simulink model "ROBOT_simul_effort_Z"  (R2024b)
settings: Solver=VariableStepAuto  StartTime=0.0  StopTime=5  RelTol=1e-3
undefined symbols (not defined in the file): a, ARRIERE_Defaut_sldprt, avant01_Defaut_sldprt, avant02_Defaut_sldprt, avant03_Defaut_sldprt, avant1_Defaut_sldprt, AXE, BASE_Defaut_sldprt, BIELLE, BIELLE_Defaut_sldprt, BRAS_Defaut_sldprt, bras_Defaut_sldprt, C_Realiste_sldprt, CABLE_Defaut_sldprt, cable_Defaut_sldprt, CACHE_Defaut_sldprt, CARTE, carte_Defaut_sldprt, CARTER, carter, CHC, CODEUR_Defaut_sldprt, cruciforme, cylindrique, deg, Drive, Fichiers, Fichiers_Matlab_sujetA, FIXATION, fixation_Defaut_sldprt, H, HEXAGONALE_Defaut_sldprt, joint_Defaut_sldprt, kg, m, M4, M4_Defaut_sldprt, manette1_Defaut_sldprt, manette2_Defaut_sldprt, MATLAB, Matlab, matlab_Defaut_sldprt, mm, modif, MOTEUR_Defaut_sldprt, N, NEZ_Defaut_sldprt, nom, palier, PARALLELOGRAMME_Defaut_sldprt, petite, plaque, rad, Ressort, Rondelle, ROTOR_Defaut_sldprt, s, SET, simple, socle_Defaut_sldprt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
libraries: sm_lib x463, fl_lib x45, nesl_utility x27, simulink x2
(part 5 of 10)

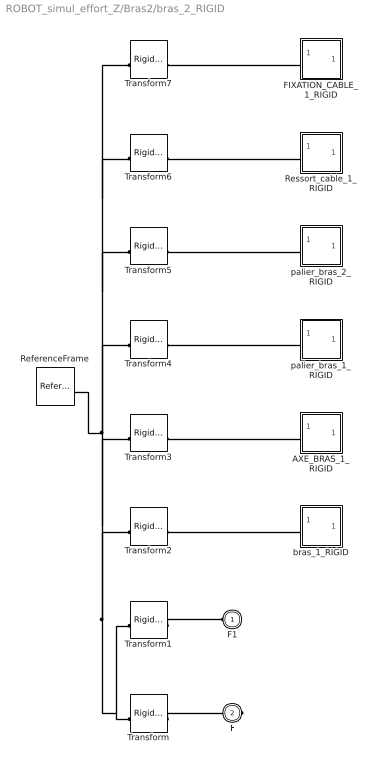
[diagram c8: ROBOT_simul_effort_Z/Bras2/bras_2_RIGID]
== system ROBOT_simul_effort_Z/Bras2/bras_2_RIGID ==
  AXE_BRAS_1_RIGID : Subsystem
  FIXATION_CABLE_1_RIGID : Subsystem
  ReferenceFrame : sm_lib/Frames and Transforms/Reference Frame
  Ressort_cable_1_RIGID : Subsystem
  Transform : sm_lib/Frames and Transforms/Rigid Transform  RotationMethod=ArbitraryAxis  FollAlignAxisA=+X  BaseAlignAxisA=+Y  FollAlignAxisB=+Y  BaseAlignAxisB=+Z  RotationStandardAxis=+Z  RotationAngle=2.0943951023931953  RotationAngleUnits=rad  RotationArbitraryAxis=[0.57735026918962584 0.57735026918962562 0.57735026918962584]  RotationSequenceAxes=FollowerAxes  RotationSequence=XYX  RotationSequenceAngles=[0 0 0]  RotationSequenceAnglesUnits=deg  RotationMatrix=[1 0 0; 0 1 0; 0 0 1]  Quaternion=[1 0 0 0]  TranslationMethod=Cartesian  TranslationCartesianOffset=[-176.59192436800635 99.825618202078147 -20.98098974470366]  TranslationCartesianOffsetUnits=mm  TranslationStandardAxis=+Z  TranslationStandardOffset=0  TranslationStandardOffsetUnits=mm  TranslationROffset=0  TranslationROffsetUnits=m  TranslationThetaOffset=0  TranslationThetaOffsetUnits=deg  TranslationZOffset=0  TranslationZOffsetUnits=m
  Transform1 : sm_lib/Frames and Transforms/Rigid Transform  RotationMethod=ArbitraryAxis  FollAlignAxisA=+X  BaseAlignAxisA=+Y  FollAlignAxisB=+Y  BaseAlignAxisB=+Z  RotationStandardAxis=+Z  RotationAngle=2.0943951023931948  RotationAngleUnits=rad  RotationArbitraryAxis=[0.57735026918962573 0.57735026918962562 0.57735026918962595]  RotationSequenceAxes=FollowerAxes  RotationSequence=XYX  RotationSequenceAngles=[0 0 0]  RotationSequenceAnglesUnits=deg  RotationMatrix=[1 0 0; 0 1 0; 0 0 1]  Quaternion=[1 0 0 0]  TranslationMethod=Cartesian  TranslationCartesianOffset=[-252.36832285678628 39.825618202076186 -20.980989744713362]  TranslationCartesianOffsetUnits=mm  TranslationStandardAxis=+Z  TranslationStandardOffset=0  TranslationStandardOffsetUnits=mm  TranslationROffset=0  TranslationROffsetUnits=m  TranslationThetaOffset=0  TranslationThetaOffsetUnits=deg  TranslationZOffset=0  TranslationZOffsetUnits=m
  Transform2 : sm_lib/Frames and Transforms/Rigid Transform  RotationMethod=ArbitraryAxis  FollAlignAxisA=+X  BaseAlignAxisA=+Y  FollAlignAxisB=+Y  BaseAlignAxisB=+Z  RotationStandardAxis=+Z  RotationAngle=1.5707963267948968  RotationAngleUnits=rad  RotationArbitraryAxis=[9.841111005584301e-17 -1 -9.841111005584301e-17]  RotationSequenceAxes=FollowerAxes  RotationSequence=XYX  RotationSequenceAngles=[0 0 0]  RotationSequenceAnglesUnits=deg  RotationMatrix=[1 0 0; 0 1 0; 0 0 1]  Quaternion=[1 0 0 0]  TranslationMethod=Cartesian  TranslationCartesianOffset=[-166.59192436800635 39.825618202078161 -20.98098974470367]  TranslationCartesianOffsetUnits=mm  TranslationStandardAxis=+Z  TranslationStandardOffset=0  TranslationStandardOffsetUnits=mm  TranslationROffset=0  TranslationROffsetUnits=m  TranslationThetaOffset=0  TranslationThetaOffsetUnits=deg  TranslationZOffset=0  TranslationZOffsetUnits=m
  Transform3 : sm_lib/Frames and Transforms/Rigid Transform  RotationMethod=ArbitraryAxis  FollAlignAxisA=+X  BaseAlignAxisA=+Y  FollAlignAxisB=+Y  BaseAlignAxisB=+Z  RotationStandardAxis=+Z  RotationAngle=1.5707963267948968  RotationAngleUnits=rad  RotationArbitraryAxis=[-9.841111005584301e-17 1 -9.841111005584301e-17]  RotationSequenceAxes=FollowerAxes  RotationSequence=XYX  RotationSequenceAngles=[0 0 0]  RotationSequenceAnglesUnits=deg  RotationMatrix=[1 0 0; 0 1 0; 0 0 1]  Quaternion=[1 0 0 0]  TranslationMethod=Cartesian  TranslationCartesianOffset=[-166.59192436800635 39.825618202078161 -20.98098974470367]  TranslationCartesianOffsetUnits=mm  TranslationStandardAxis=+Z  TranslationStandardOffset=0  TranslationStandardOffsetUnits=mm  TranslationROffset=0  TranslationROffsetUnits=m  TranslationThetaOffset=0  TranslationThetaOffsetUnits=deg  TranslationZOffset=0  TranslationZOffsetUnits=m
  Transform4 : sm_lib/Frames and Transforms/Rigid Transform  RotationMethod=None  FollAlignAxisA=+X  BaseAlignAxisA=+Y  FollAlignAxisB=+Y  BaseAlignAxisB=+Z  RotationStandardAxis=+Z  RotationAngle=0  RotationAngleUnits=deg  RotationArbitraryAxis=[0 0 1]  RotationSequenceAxes=FollowerAxes  RotationSequence=XYX  RotationSequenceAngles=[0 0 0]  RotationSequenceAnglesUnits=deg  RotationMatrix=[1 0 0; 0 1 0; 0 0 1]  Quaternion=[1 0 0 0]  TranslationMethod=None  TranslationCartesianOffset=[0 0 0]  TranslationCartesianOffsetUnits=m  TranslationStandardAxis=+Z  TranslationStandardOffset=0  TranslationStandardOffsetUnits=m  TranslationROffset=0  TranslationROffsetUnits=m  TranslationThetaOffset=0  TranslationThetaOffsetUnits=deg  TranslationZOffset=0  TranslationZOffsetUnits=m
  Transform5 : sm_lib/Frames and Transforms/Rigid Transform  RotationMethod=ArbitraryAxis  FollAlignAxisA=+X  BaseAlignAxisA=+Y  FollAlignAxisB=+Y  BaseAlignAxisB=+Z  RotationStandardAxis=+Z  RotationAngle=3.1415926535897931  RotationAngleUnits=rad  RotationArbitraryAxis=[5.9196876012963212e-17 0.83121877946981937 -0.55594544755461739]  RotationSequenceAxes=FollowerAxes  RotationSequence=XYX  RotationSequenceAngles=[0 0 0]  RotationSequenceAnglesUnits=deg  RotationMatrix=[1 0 0; 0 1 0; 0 0 1]  Quaternion=[1 0 0 0]  TranslationMethod=Cartesian  TranslationCartesianOffset=[-333.18384873601269 5.2270863233389981 7.8152493791980318]  TranslationCartesianOffsetUnits=mm  TranslationStandardAxis=+Z  TranslationStandardOffset=0  TranslationStandardOffsetUnits=mm  TranslationROffset=0  TranslationROffsetUnits=m  TranslationThetaOffset=0  TranslationThetaOffsetUnits=deg  TranslationZOffset=0  TranslationZOffsetUnits=m
  Transform6 : sm_lib/Frames and Transforms/Rigid Transform  RotationMethod=ArbitraryAxis  FollAlignAxisA=+X  BaseAlignAxisA=+Y  FollAlignAxisB=+Y  BaseAlignAxisB=+Z  RotationStandardAxis=+Z  RotationAngle=1.5707963267948968  RotationAngleUnits=rad  RotationArbitraryAxis=[1 -9.841111005584301e-17 9.8411110055842801e-17]  RotationSequenceAxes=FollowerAxes  RotationSequence=XYX  RotationSequenceAngles=[0 0 0]  RotationSequenceAnglesUnits=deg  RotationMatrix=[1 0 0; 0 1 0; 0 0 1]  Quaternion=[1 0 0 0]  TranslationMethod=Cartesian  TranslationCartesianOffset=[-166.59192436800635 17.1829411352671 -24.980989744703674]  TranslationCartesianOffsetUnits=mm  TranslationStandardAxis=+Z  TranslationStandardOffset=0  TranslationStandardOffsetUnits=mm  TranslationROffset=0  TranslationROffsetUnits=m  TranslationThetaOffset=0  TranslationThetaOffsetUnits=deg  TranslationZOffset=0  TranslationZOffsetUnits=m
  Transform7 : sm_lib/Frames and Transforms/Rigid Transform  RotationMethod=ArbitraryAxis  FollAlignAxisA=+X  BaseAlignAxisA=+Y  FollAlignAxisB=+Y  BaseAlignAxisB=+Z  RotationStandardAxis=+Z  RotationAngle=1.0159852938148253  RotationAngleUnits=rad  RotationArbitraryAxis=[-1 0 -1.1577777653628589e-16]  RotationSequenceAxes=FollowerAxes  RotationSequence=XYX  RotationSequenceAngles=[0 0 0]  RotationSequenceAnglesUnits=deg  RotationMatrix=[1 0 0; 0 1 0; 0 0 1]  Quaternion=[1 0 0 0]  TranslationMethod=Cartesian  TranslationCartesianOffset=[-172.59192436800635 90.586314327933934 3.4188407632840172]  TranslationCartesianOffsetUnits=mm  TranslationStandardAxis=+Z  TranslationStandardOffset=0  TranslationStandardOffsetUnits=mm  TranslationROffset=0  TranslationROffsetUnits=m  TranslationThetaOffset=0  TranslationThetaOffsetUnits=deg  TranslationZOffset=0  TranslationZOffsetUnits=m
  bras_1_RIGID : Subsystem
  palier_bras_1_RIGID : Subsystem
  palier_bras_2_RIGID : Subsystem
  F1 : PMIOPort  Side=Left
  F : PMIOPort  Port=2  Side=Right
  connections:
  Transform/LConn1 -- ReferenceFrame/RConn1 -- Transform6/LConn1 -- Transform7/LConn1 -- Transform5/LConn1 -- Transform4/LConn1 -- Transform3/LConn1 -- Transform2/LConn1 -- Transform1/LConn1
  Transform/RConn1 -- F/RConn1
  Transform1/RConn1 -- F1/RConn1
  Transform2/RConn1 -- bras_1_RIGID/LConn1
  AXE_BRAS_1_RIGID/LConn1 -- Transform3/RConn1
  Transform4/RConn1 -- palier_bras_1_RIGID/LConn1
  Transform5/RConn1 -- palier_bras_2_RIGID/LConn1
  Ressort_cable_1_RIGID/LConn1 -- Transform6/RConn1
  FIXATION_CABLE_1_RIGID/LConn1 -- Transform7/RConn1

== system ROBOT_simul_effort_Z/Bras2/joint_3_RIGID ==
  AXE_BRAS_1_RIGID : Subsystem
  ReferenceFrame : sm_lib/Frames and Transforms/Reference Frame
  Transform : sm_lib/Frames and Transforms/Rigid Transform  RotationMethod=ArbitraryAxis  FollAlignAxisA=+X  BaseAlignAxisA=+Y  FollAlignAxisB=+Y  BaseAlignAxisB=+Z  RotationStandardAxis=+Z  RotationAngle=2.0943951023931953  RotationAngleUnits=rad  RotationArbitraryAxis=[0.57735026918962584 0.57735026918962584 0.57735026918962584]  RotationSequenceAxes=FollowerAxes  RotationSequence=XYX  RotationSequenceAngles=[0 0 0]  RotationSequenceAnglesUnits=deg  RotationMatrix=[1 0 0; 0 1 0; 0 0 1]  Quaternion=[1 0 0 0]  TranslationMethod=Cartesian  TranslationCartesianOffset=[-182.62772197331239 126.3991346976174 -143.1183707091507]  TranslationCartesianOffsetUnits=mm  TranslationStandardAxis=+Z  TranslationStandardOffset=0  TranslationStandardOffsetUnits=mm  TranslationROffset=0  TranslationROffsetUnits=m  TranslationThetaOffset=0  TranslationThetaOffsetUnits=deg  TranslationZOffset=0  TranslationZOffsetUnits=m
  Transform1 : sm_lib/Frames and Transforms/Rigid Transform  RotationMethod=ArbitraryAxis  FollAlignAxisA=+X  BaseAlignAxisA=+Y  FollAlignAxisB=+Y  BaseAlignAxisB=+Z  RotationStandardAxis=+Z  RotationAngle=1.9754511492118267  RotationAngleUnits=rad  RotationArbitraryAxis=[-0.53149434051907762 -0.5314943405190774 -0.65956616953296032]  RotationSequenceAxes=FollowerAxes  RotationSequence=XYX  RotationSequenceAngles=[0 0 0]  RotationSequenceAnglesUnits=deg  RotationMatrix=[1 0 0; 0 1 0; 0 0 1]  Quaternion=[1 0 0 0]  TranslationMethod=Cartesian  TranslationCartesianOffset=[-181.62772197331239 116.1902983931664 -133.8263224253264]  TranslationCartesianOffsetUnits=mm  TranslationStandardAxis=+Z  TranslationStandardOffset=0  TranslationStandardOffsetUnits=mm  TranslationROffset=0  TranslationROffsetUnits=m  TranslationThetaOffset=0  TranslationThetaOffsetUnits=deg  TranslationZOffset=0  TranslationZOffsetUnits=m
  Transform2 : sm_lib/Frames and Transforms/Rigid Transform  RotationMethod=ArbitraryAxis  FollAlignAxisA=+X  BaseAlignAxisA=+Y  FollAlignAxisB=+Y  BaseAlignAxisB=+Z  RotationStandardAxis=+Z  RotationAngle=1.9754511492118267  RotationAngleUnits=rad  RotationArbitraryAxis=[-0.53149434051907762 -0.5314943405190774 -0.65956616953296032]  RotationSequenceAxes=FollowerAxes  RotationSequence=XYX  RotationSequenceAngles=[0 0 0]  RotationSequenceAnglesUnits=deg  RotationMatrix=[1 0 0; 0 1 0; 0 0 1]  Quaternion=[1 0 0 0]  TranslationMethod=Cartesian  TranslationCartesianOffset=[-153.62772197331239 116.19029839316639 -133.82632242532642]  TranslationCartesianOffsetUnits=mm  TranslationStandardAxis=+Z  TranslationStandardOffset=0  TranslationStandardOffsetUnits=mm  TranslationROffset=0  TranslationROffsetUnits=m  TranslationThetaOffset=0  TranslationThetaOffsetUnits=deg  TranslationZOffset=0  TranslationZOffsetUnits=m
  Transform3 : sm_lib/Frames and Transforms/Rigid Transform  RotationMethod=ArbitraryAxis  FollAlignAxisA=+X  BaseAlignAxisA=+Y  FollAlignAxisB=+Y  BaseAlignAxisB=+Z  RotationStandardAxis=+Z  RotationAngle=1.7850283121554718  RotationAngleUnits=rad  RotationArbitraryAxis=[1 6.7005179906918671e-16 -7.8797744802439854e-16]  RotationSequenceAxes=FollowerAxes  RotationSequence=XYX  RotationSequenceAngles=[0 0 0]  RotationSequenceAnglesUnits=deg  RotationMatrix=[1 0 0; 0 1 0; 0 0 1]  Quaternion=[1 0 0 0]  TranslationMethod=Cartesian  TranslationCartesianOffset=[-167.62772197331242 128.09991096385988 -150.93549038919826]  TranslationCartesianOffsetUnits=mm  TranslationStandardAxis=+Z  TranslationStandardOffset=0  TranslationStandardOffsetUnits=mm  TranslationROffset=0  TranslationROffsetUnits=m  TranslationThetaOffset=0  TranslationThetaOffsetUnits=deg  TranslationZOffset=0  TranslationZOffsetUnits=m
  Transform4 : sm_lib/Frames and Transforms/Rigid Transform  RotationMethod=ArbitraryAxis  FollAlignAxisA=+X  BaseAlignAxisA=+Y  FollAlignAxisB=+Y  BaseAlignAxisB=+Z  RotationStandardAxis=+Z  RotationAngle=1.5707963267948968  RotationAngleUnits=rad  RotationArbitraryAxis=[8.0498418078381935e-17 -1 8.0498418078381935e-17]  RotationSequenceAxes=FollowerAxes  RotationSequence=XYX  RotationSequenceAngles=[0 0 0]  RotationSequenceAnglesUnits=deg  RotationMatrix=[1 0 0; 0 1 0; 0 0 1]  Quaternion=[1 0 0 0]  TranslationMethod=Cartesian  TranslationCartesianOffset=[-167.62772197331239 126.3991346976174 -143.1183707091507]  TranslationCartesianOffsetUnits=mm  TranslationStandardAxis=+Z  TranslationStandardOffset=0  TranslationStandardOffsetUnits=mm  TranslationROffset=0  TranslationROffsetUnits=m  TranslationThetaOffset=0  TranslationThetaOffsetUnits=deg  TranslationZOffset=0  TranslationZOffsetUnits=m
  joint_1_RIGID : Subsystem
  F2 : PMIOPort  Side=Left
  F : PMIOPort  Port=2  Side=Right
  F1 : PMIOPort  Port=3  Side=Left
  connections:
  Transform/LConn1 -- ReferenceFrame/RConn1 -- Transform3/LConn1 -- Transform4/LConn1 -- Transform2/LConn1 -- Transform1/LConn1
  Transform/RConn1 -- F/RConn1
  Transform1/RConn1 -- F1/RConn1
  Transform2/RConn1 -- F2/RConn1
  Transform3/RConn1 -- joint_1_RIGID/LConn1
  AXE_BRAS_1_RIGID/LConn1 -- Transform4/RConn1

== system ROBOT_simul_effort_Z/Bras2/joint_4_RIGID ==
  AXE_BRAS_1_RIGID : Subsystem
  ReferenceFrame : sm_lib/Frames and Transforms/Reference Frame
  Transform : sm_lib/Frames and Transforms/Rigid Transform  RotationMethod=ArbitraryAxis  FollAlignAxisA=+X  BaseAlignAxisA=+Y  FollAlignAxisB=+Y  BaseAlignAxisB=+Z  RotationStandardAxis=+Z  RotationAngle=2.0943951023931962  RotationAngleUnits=rad  RotationArbitraryAxis=[0.5773502691896254 0.57735026918962584 0.57735026918962595]  RotationSequenceAxes=FollowerAxes  RotationSequence=XYX  RotationSequenceAngles=[0 0 0]  RotationSequenceAnglesUnits=deg  RotationMatrix=[1 0 0; 0 1 0; 0 0 1]  Quaternion=[1 0 0 0]  TranslationMethod=Cartesian  TranslationCartesianOffset=[-177.62772197331228 126.39913469764599 -143.11837070916687]  TranslationCartesianOffsetUnits=mm  TranslationStandardAxis=+Z  TranslationStandardOffset=0  TranslationStandardOffsetUnits=mm  TranslationROffset=0  TranslationROffsetUnits=m  TranslationThetaOffset=0  TranslationThetaOffsetUnits=deg  TranslationZOffset=0  TranslationZOffsetUnits=m
  Transform1 : sm_lib/Frames and Transforms/Rigid Transform  RotationMethod=ArbitraryAxis  FollAlignAxisA=+X  BaseAlignAxisA=+Y  FollAlignAxisB=+Y  BaseAlignAxisB=+Z  RotationStandardAxis=+Z  RotationAngle=1.9754511492118263  RotationAngleUnits=rad  RotationArbitraryAxis=[-0.53149434051907762 -0.53149434051907762 -0.6595661695329601]  RotationSequenceAxes=FollowerAxes  RotationSequence=XYX  RotationSequenceAngles=[0 0 0]  RotationSequenceAnglesUnits=deg  RotationMatrix=[1 0 0; 0 1 0; 0 0 1]  Quaternion=[1 0 0 0]  TranslationMethod=Cartesian  TranslationCartesianOffset=[-181.6277219733183 116.19029839316549 -133.82632242532227]  TranslationCartesianOffsetUnits=mm  TranslationStandardAxis=+Z  TranslationStandardOffset=0  TranslationStandardOffsetUnits=mm  TranslationROffset=0  TranslationROffsetUnits=m  TranslationThetaOffset=0  TranslationThetaOffsetUnits=deg  TranslationZOffset=0  TranslationZOffsetUnits=m
  Transform2 : sm_lib/Frames and Transforms/Rigid Transform  RotationMethod=ArbitraryAxis  FollAlignAxisA=+X  BaseAlignAxisA=+Y  FollAlignAxisB=+Y  BaseAlignAxisB=+Z  RotationStandardAxis=+Z  RotationAngle=2.2221940470110662  RotationAngleUnits=rad  RotationArbitraryAxis=[0.61437017396792992 -0.61437017396793137 0.49507431631748922]  RotationSequenceAxes=FollowerAxes  RotationSequence=XYX  RotationSequenceAngles=[0 0 0]  RotationSequenceAnglesUnits=deg  RotationMatrix=[1 0 0; 0 1 0; 0 0 1]  Quaternion=[1 0 0 0]  TranslationMethod=Cartesian  TranslationCartesianOffset=[-153.62772197331839 131.82453775326127 -130.42476989284023]  TranslationCartesianOffsetUnits=mm  TranslationStandardAxis=+Z  TranslationStandardOffset=0  TranslationStandardOffsetUnits=mm  TranslationROffset=0  TranslationROffsetUnits=m  TranslationThetaOffset=0  TranslationThetaOffsetUnits=deg  TranslationZOffset=0  TranslationZOffsetUnits=m
  Transform3 : sm_lib/Frames and Transforms/Rigid Transform  RotationMethod=ArbitraryAxis  FollAlignAxisA=+X  BaseAlignAxisA=+Y  FollAlignAxisB=+Y  BaseAlignAxisB=+Z  RotationStandardAxis=+Z  RotationAngle=1.785028312155472  RotationAngleUnits=rad  RotationArbitraryAxis=[1 8.8696087027513098e-16 -7.493533857789905e-16]  RotationSequenceAxes=FollowerAxes  RotationSequence=XYX  RotationSequenceAngles=[0 0 0]  RotationSequenceAnglesUnits=deg  RotationMatrix=[1 0 0; 0 1 0; 0 0 1]  Quaternion=[1 0 0 0]  TranslationMethod=Cartesian  TranslationCartesianOffset=[-167.62772197331242 128.09991096385986 -150.93549038919815]  TranslationCartesianOffsetUnits=mm  TranslationStandardAxis=+Z  TranslationStandardOffset=0  TranslationStandardOffsetUnits=mm  TranslationROffset=0  TranslationROffsetUnits=m  TranslationThetaOffset=0  TranslationThetaOffsetUnits=deg  TranslationZOffset=0  TranslationZOffsetUnits=m
  Transform4 : sm_lib/Frames and Transforms/Rigid Transform  RotationMethod=ArbitraryAxis  FollAlignAxisA=+X  BaseAlignAxisA=+Y  FollAlignAxisB=+Y  BaseAlignAxisB=+Z  RotationStandardAxis=+Z  RotationAngle=1.570796326794897  RotationAngleUnits=rad  RotationArbitraryAxis=[-0 -1 -0]  RotationSequenceAxes=FollowerAxes  RotationSequence=XYX  RotationSequenceAngles=[0 0 0]  RotationSequenceAnglesUnits=deg  RotationMatrix=[1 0 0; 0 1 0; 0 0 1]  Quaternion=[1 0 0 0]  TranslationMethod=Cartesian  TranslationCartesianOffset=[-167.62772197331239 126.39913469761737 -143.11837070915061]  TranslationCartesianOffsetUnits=mm  TranslationStandardAxis=+Z  TranslationStandardOffset=0  TranslationStandardOffsetUnits=mm  TranslationROffset=0  TranslationROffsetUnits=m  TranslationThetaOffset=0  TranslationThetaOffsetUnits=deg  TranslationZOffset=0  TranslationZOffsetUnits=m
  joint_1_RIGID : Subsystem
  F2 : PMIOPort  Side=Right
  F1 : PMIOPort  Port=2  Side=Right
  F : PMIOPort  Port=3  Side=Left
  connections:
  Transform/LConn1 -- ReferenceFrame/RConn1 -- Transform3/LConn1 -- Transform4/LConn1 -- Transform2/LConn1 -- Transform1/LConn1
  Transform/RConn1 -- F/RConn1
  Transform1/RConn1 -- F1/RConn1
  Transform2/RConn1 -- F2/RConn1
  Transform3/RConn1 -- joint_1_RIGID/LConn1
  AXE_BRAS_1_RIGID/LConn1 -- Transform4/RConn1

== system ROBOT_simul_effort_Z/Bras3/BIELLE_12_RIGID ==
  AXE_BIELLE_1_RIGID : Subsystem
  AXE_BIELLE_2_RIGID : Subsystem
  BIELLE_PARALLELOGRAMME_1_RIGID : Subsystem
  ReferenceFrame : sm_lib/Frames and Transforms/Reference Frame
  Transform : sm_lib/Frames and Transforms/Rigid Transform  RotationMethod=ArbitraryAxis  FollAlignAxisA=+X  BaseAlignAxisA=+Y  FollAlignAxisB=+Y  BaseAlignAxisB=+Z  RotationStandardAxis=+Z  RotationAngle=2.0943951023931953  RotationAngleUnits=rad  RotationArbitraryAxis=[0.57735026918962584 -0.57735026918962584 0.57735026918962584]  RotationSequenceAxes=FollowerAxes  RotationSequence=XYX  RotationSequenceAngles=[0 0 0]  RotationSequenceAnglesUnits=deg  RotationMatrix=[1 0 0; 0 1 0; 0 0 1]  Quaternion=[1 0 0 0]  TranslationMethod=Cartesian  TranslationCartesianOffset=[-181.12877100136717 12.999999999999996 -3.249999999999996]  TranslationCartesianOffsetUnits=mm  TranslationStandardAxis=+Z  TranslationStandardOffset=0  TranslationStandardOffsetUnits=mm  TranslationROffset=0  TranslationROffsetUnits=m  TranslationThetaOffset=0  TranslationThetaOffsetUnits=deg  TranslationZOffset=0  TranslationZOffsetUnits=m
  Transform1 : sm_lib/Frames and Transforms/Rigid Transform  RotationMethod=ArbitraryAxis  FollAlignAxisA=+X  BaseAlignAxisA=+Y  FollAlignAxisB=+Y  BaseAlignAxisB=+Z  RotationStandardAxis=+Z  RotationAngle=2.0943951023931957  RotationAngleUnits=rad  RotationArbitraryAxis=[0.57735026918962573 -0.57735026918962573 0.57735026918962562]  RotationSequenceAxes=FollowerAxes  RotationSequence=XYX  RotationSequenceAngles=[0 0 0]  RotationSequenceAnglesUnits=deg  RotationMatrix=[1 0 0; 0 1 0; 0 0 1]  Quaternion=[1 0 0 0]  TranslationMethod=Cartesian  TranslationCartesianOffset=[-181.1287710013672 12.999999999999963 -105.75000000000004]  TranslationCartesianOffsetUnits=mm  TranslationStandardAxis=+Z  TranslationStandardOffset=0  TranslationStandardOffsetUnits=mm  TranslationROffset=0  TranslationROffsetUnits=m  TranslationThetaOffset=0  TranslationThetaOffsetUnits=deg  TranslationZOffset=0  TranslationZOffsetUnits=m
  Transform2 : sm_lib/Frames and Transforms/Rigid Transform  RotationMethod=ArbitraryAxis  FollAlignAxisA=+X  BaseAlignAxisA=+Y  FollAlignAxisB=+Y  BaseAlignAxisB=+Z  RotationStandardAxis=+Z  RotationAngle=3.1415926535897931  RotationAngleUnits=rad  RotationArbitraryAxis=[-0.70710678118654746 0.70710678118654757 0]  RotationSequenceAxes=FollowerAxes  RotationSequence=XYX  RotationSequenceAngles=[0 0 0]  RotationSequenceAnglesUnits=deg  RotationMatrix=[1 0 0; 0 1 0; 0 0 1]  Quaternion=[1 0 0 0]  TranslationMethod=Cartesian  TranslationCartesianOffset=[-178.12877100136717 4.9999999999999902 -54.500000000000021]  TranslationCartesianOffsetUnits=mm  TranslationStandardAxis=+Z  TranslationStandardOffset=0  TranslationStandardOffsetUnits=mm  TranslationROffset=0  TranslationROffsetUnits=m  TranslationThetaOffset=0  TranslationThetaOffsetUnits=deg  TranslationZOffset=0  TranslationZOffsetUnits=m
  Transform3 : sm_lib/Frames and Transforms/Rigid Transform  RotationMethod=ArbitraryAxis  FollAlignAxisA=+X  BaseAlignAxisA=+Y  FollAlignAxisB=+Y  BaseAlignAxisB=+Z  RotationStandardAxis=+Z  RotationAngle=1.7602050674842991  RotationAngleUnits=rad  RotationArbitraryAxis=[-0.82650316451596495 -0.39805308631204944 -0.39805308631204944]  RotationSequenceAxes=FollowerAxes  RotationSequence=XYX  RotationSequenceAngles=[0 0 0]  RotationSequenceAnglesUnits=deg  RotationMatrix=[1 0 0; 0 1 0; 0 0 1]  Quaternion=[1 0 0 0]  TranslationMethod=Cartesian  TranslationCartesianOffset=[-181.1287710013672 4.9999999999999627 -105.75000000000004]  TranslationCartesianOffsetUnits=mm  TranslationStandardAxis=+Z  TranslationStandardOffset=0  TranslationStandardOffsetUnits=mm  TranslationROffset=0  TranslationROffsetUnits=m  TranslationThetaOffset=0  TranslationThetaOffsetUnits=deg  TranslationZOffset=0  TranslationZOffsetUnits=m
  Transform4 : sm_lib/Frames and Transforms/Rigid Transform  RotationMethod=ArbitraryAxis  FollAlignAxisA=+X  BaseAlignAxisA=+Y  FollAlignAxisB=+Y  BaseAlignAxisB=+Z  RotationStandardAxis=+Z  RotationAngle=1.7602050674842997  RotationAngleUnits=rad  RotationArbitraryAxis=[-0.82650316451596506 -0.39805308631204933 -0.39805308631204939]  RotationSequenceAxes=FollowerAxes  RotationSequence=XYX  RotationSequenceAngles=[0 0 0]  RotationSequenceAnglesUnits=deg  RotationMatrix=[1 0 0; 0 1 0; 0 0 1]  Quaternion=[1 0 0 0]  TranslationMethod=Cartesian  TranslationCartesianOffset=[-181.12877100136717 4.9999999999999902 -3.249999999999996]  TranslationCartesianOffsetUnits=mm  TranslationStandardAxis=+Z  TranslationStandardOffset=0  TranslationStandardOffsetUnits=mm  TranslationROffset=0  TranslationROffsetUnits=m  TranslationThetaOffset=0  TranslationThetaOffsetUnits=deg  TranslationZOffset=0  TranslationZOffsetUnits=m
  F1 : PMIOPort  Side=Left
  F : PMIOPort  Port=2  Side=Right
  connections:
  Transform/LConn1 -- ReferenceFrame/RConn1 -- Transform3/LConn1 -- Transform4/LConn1 -- Transform2/LConn1 -- Transform1/LConn1
  Transform/RConn1 -- F/RConn1
  Transform1/RConn1 -- F1/RConn1
  BIELLE_PARALLELOGRAMME_1_RIGID/LConn1 -- Transform2/RConn1
  AXE_BIELLE_1_RIGID/LConn1 -- Transform3/RConn1
  AXE_BIELLE_2_RIGID/LConn1 -- Transform4/RConn1

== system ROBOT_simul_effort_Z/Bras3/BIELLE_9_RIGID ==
  AXE_BIELLE_1_RIGID : Subsystem
  AXE_BIELLE_2_RIGID : Subsystem
  BIELLE_PARALLELOGRAMME_1_RIGID : Subsystem
  ReferenceFrame : sm_lib/Frames and Transforms/Reference Frame
  Transform : sm_lib/Frames and Transforms/Rigid Transform  RotationMethod=ArbitraryAxis  FollAlignAxisA=+X  BaseAlignAxisA=+Y  FollAlignAxisB=+Y  BaseAlignAxisB=+Z  RotationStandardAxis=+Z  RotationAngle=2.0943951023931957  RotationAngleUnits=rad  RotationArbitraryAxis=[0.57735026918962573 -0.57735026918962573 0.57735026918962562]  RotationSequenceAxes=FollowerAxes  RotationSequence=XYX  RotationSequenceAngles=[0 0 0]  RotationSequenceAnglesUnits=deg  RotationMatrix=[1 0 0; 0 1 0; 0 0 1]  Quaternion=[1 0 0 0]  TranslationMethod=Cartesian  TranslationCartesianOffset=[-181.12877100136723 12.999999999999982 -105.75000000000001]  TranslationCartesianOffsetUnits=mm  TranslationStandardAxis=+Z  TranslationStandardOffset=0  TranslationStandardOffsetUnits=mm  TranslationROffset=0  TranslationROffsetUnits=m  TranslationThetaOffset=0  TranslationThetaOffsetUnits=deg  TranslationZOffset=0  TranslationZOffsetUnits=m
  Transform1 : sm_lib/Frames and Transforms/Rigid Transform  RotationMethod=ArbitraryAxis  FollAlignAxisA=+X  BaseAlignAxisA=+Y  FollAlignAxisB=+Y  BaseAlignAxisB=+Z  RotationStandardAxis=+Z  RotationAngle=2.0943951023931957  RotationAngleUnits=rad  RotationArbitraryAxis=[0.57735026918962584 -0.57735026918962573 0.57735026918962573]  RotationSequenceAxes=FollowerAxes  RotationSequence=XYX  RotationSequenceAngles=[0 0 0]  RotationSequenceAnglesUnits=deg  RotationMatrix=[1 0 0; 0 1 0; 0 0 1]  Quaternion=[1 0 0 0]  TranslationMethod=Cartesian  TranslationCartesianOffset=[-181.12877100136717 13.000000000000004 -3.2500000000000151]  TranslationCartesianOffsetUnits=mm  TranslationStandardAxis=+Z  TranslationStandardOffset=0  TranslationStandardOffsetUnits=mm  TranslationROffset=0  TranslationROffsetUnits=m  TranslationThetaOffset=0  TranslationThetaOffsetUnits=deg  TranslationZOffset=0  TranslationZOffsetUnits=m
  Transform2 : sm_lib/Frames and Transforms/Rigid Transform  RotationMethod=ArbitraryAxis  FollAlignAxisA=+X  BaseAlignAxisA=+Y  FollAlignAxisB=+Y  BaseAlignAxisB=+Z  RotationStandardAxis=+Z  RotationAngle=3.1415926535897931  RotationAngleUnits=rad  RotationArbitraryAxis=[0.70710678118654746 -0.70710678118654757 3.9252311467094379e-17]  RotationSequenceAxes=FollowerAxes  RotationSequence=XYX  RotationSequenceAngles=[0 0 0]  RotationSequenceAnglesUnits=deg  RotationMatrix=[1 0 0; 0 1 0; 0 0 1]  Quaternion=[1 0 0 0]  TranslationMethod=Cartesian  TranslationCartesianOffset=[-178.12877100136717 5.0000000000000044 -54.500000000000021]  TranslationCartesianOffsetUnits=mm  TranslationStandardAxis=+Z  TranslationStandardOffset=0  TranslationStandardOffsetUnits=mm  TranslationROffset=0  TranslationROffsetUnits=m  TranslationThetaOffset=0  TranslationThetaOffsetUnits=deg  TranslationZOffset=0  TranslationZOffsetUnits=m
  Transform3 : sm_lib/Frames and Transforms/Rigid Transform  RotationMethod=ArbitraryAxis  FollAlignAxisA=+X  BaseAlignAxisA=+Y  FollAlignAxisB=+Y  BaseAlignAxisB=+Z  RotationStandardAxis=+Z  RotationAngle=1.7602050674842991  RotationAngleUnits=rad  RotationArbitraryAxis=[-0.82650316451596495 -0.39805308631204944 -0.39805308631204944]  RotationSequenceAxes=FollowerAxes  RotationSequence=XYX  RotationSequenceAngles=[0 0 0]  RotationSequenceAnglesUnits=deg  RotationMatrix=[1 0 0; 0 1 0; 0 0 1]  Quaternion=[1 0 0 0]  TranslationMethod=Cartesian  TranslationCartesianOffset=[-181.12877100136723 4.9999999999999902 -105.75000000000001]  TranslationCartesianOffsetUnits=mm  TranslationStandardAxis=+Z  TranslationStandardOffset=0  TranslationStandardOffsetUnits=mm  TranslationROffset=0  TranslationROffsetUnits=m  TranslationThetaOffset=0  TranslationThetaOffsetUnits=deg  TranslationZOffset=0  TranslationZOffsetUnits=m
  Transform4 : sm_lib/Frames and Transforms/Rigid Transform  RotationMethod=ArbitraryAxis  FollAlignAxisA=+X  BaseAlignAxisA=+Y  FollAlignAxisB=+Y  BaseAlignAxisB=+Z  RotationStandardAxis=+Z  RotationAngle=1.7602050674842993  RotationAngleUnits=rad  RotationArbitraryAxis=[-0.82650316451596495 -0.39805308631204939 -0.39805308631204939]  RotationSequenceAxes=FollowerAxes  RotationSequence=XYX  RotationSequenceAngles=[0 0 0]  RotationSequenceAnglesUnits=deg  RotationMatrix=[1 0 0; 0 1 0; 0 0 1]  Quaternion=[1 0 0 0]  TranslationMethod=Cartesian  TranslationCartesianOffset=[-181.12877100136717 5.0000000000000044 -3.2500000000000169]  TranslationCartesianOffsetUnits=mm  TranslationStandardAxis=+Z  TranslationStandardOffset=0  TranslationStandardOffsetUnits=mm  TranslationROffset=0  TranslationROffsetUnits=m  TranslationThetaOffset=0  TranslationThetaOffsetUnits=deg  TranslationZOffset=0  TranslationZOffsetUnits=m
  F1 : PMIOPort  Side=Left
  F : PMIOPort  Port=2  Side=Right
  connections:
  Transform/LConn1 -- ReferenceFrame/RConn1 -- Transform3/LConn1 -- Transform4/LConn1 -- Transform2/LConn1 -- Transform1/LConn1
  Transform/RConn1 -- F/RConn1
  Transform1/RConn1 -- F1/RConn1
  BIELLE_PARALLELOGRAMME_1_RIGID/LConn1 -- Transform2/RConn1
  AXE_BIELLE_1_RIGID/LConn1 -- Transform3/RConn1
  AXE_BIELLE_2_RIGID/LConn1 -- Transform4/RConn1

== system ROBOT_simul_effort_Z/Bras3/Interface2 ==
  Angular Velocity Source : fl_lib/Mechanical/Mechanical Sources/Ideal Angular Velocity Source
  Torque Sensor : fl_lib/Mechanical/Mechanical Sensors/Ideal Torque Sensor
  C : PMIOPort  Side=Left
  T : PMIOPort  Port=2  Side=Right
  w : PMIOPort  Port=3  Side=Right
  R : PMIOPort  Port=4  Side=Left
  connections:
  R/RConn1 -- Angular Velocity Source/LConn1
  Torque Sensor/LConn1 -- Angular Velocity Source/RConn2
  Torque Sensor/RConn2 -- T/RConn1
  C/RConn1 -- Torque Sensor/RConn1
  Angular Velocity Source/RConn1 -- w/RConn1

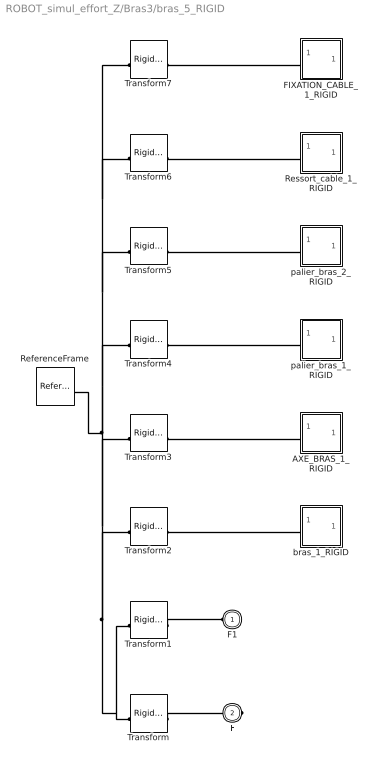
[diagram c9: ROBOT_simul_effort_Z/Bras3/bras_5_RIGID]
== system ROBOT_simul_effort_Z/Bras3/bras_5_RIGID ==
  AXE_BRAS_1_RIGID : Subsystem
  FIXATION_CABLE_1_RIGID : Subsystem
  ReferenceFrame : sm_lib/Frames and Transforms/Reference Frame
  Ressort_cable_1_RIGID : Subsystem
  Transform : sm_lib/Frames and Transforms/Rigid Transform  RotationMethod=ArbitraryAxis  FollAlignAxisA=+X  BaseAlignAxisA=+Y  FollAlignAxisB=+Y  BaseAlignAxisB=+Z  RotationStandardAxis=+Z  RotationAngle=2.0943951023931953  RotationAngleUnits=rad  RotationArbitraryAxis=[0.57735026918962584 0.57735026918962584 0.57735026918962584]  RotationSequenceAxes=FollowerAxes  RotationSequence=XYX  RotationSequenceAngles=[0 0 0]  RotationSequenceAnglesUnits=deg  RotationMatrix=[1 0 0; 0 1 0; 0 0 1]  Quaternion=[1 0 0 0]  TranslationMethod=Cartesian  TranslationCartesianOffset=[-176.59192436800632 99.825618202078189 -20.980989744703674]  TranslationCartesianOffsetUnits=mm  TranslationStandardAxis=+Z  TranslationStandardOffset=0  TranslationStandardOffsetUnits=mm  TranslationROffset=0  TranslationROffsetUnits=m  TranslationThetaOffset=0  TranslationThetaOffsetUnits=deg  TranslationZOffset=0  TranslationZOffsetUnits=m
  Transform1 : sm_lib/Frames and Transforms/Rigid Transform  RotationMethod=ArbitraryAxis  FollAlignAxisA=+X  BaseAlignAxisA=+Y  FollAlignAxisB=+Y  BaseAlignAxisB=+Z  RotationStandardAxis=+Z  RotationAngle=2.0943951023931962  RotationAngleUnits=rad  RotationArbitraryAxis=[0.57735026918962562 0.57735026918962595 0.57735026918962573]  RotationSequenceAxes=FollowerAxes  RotationSequence=XYX  RotationSequenceAngles=[0 0 0]  RotationSequenceAnglesUnits=deg  RotationMatrix=[1 0 0; 0 1 0; 0 0 1]  Quaternion=[1 0 0 0]  TranslationMethod=Cartesian  TranslationCartesianOffset=[-252.36832285678696 39.82561820208025 -20.980989744694625]  TranslationCartesianOffsetUnits=mm  TranslationStandardAxis=+Z  TranslationStandardOffset=0  TranslationStandardOffsetUnits=mm  TranslationROffset=0  TranslationROffsetUnits=m  TranslationThetaOffset=0  TranslationThetaOffsetUnits=deg  TranslationZOffset=0  TranslationZOffsetUnits=m
  Transform2 : sm_lib/Frames and Transforms/Rigid Transform  RotationMethod=ArbitraryAxis  FollAlignAxisA=+X  BaseAlignAxisA=+Y  FollAlignAxisB=+Y  BaseAlignAxisB=+Z  RotationStandardAxis=+Z  RotationAngle=1.5707963267948968  RotationAngleUnits=rad  RotationArbitraryAxis=[-0 -1 -0]  RotationSequenceAxes=FollowerAxes  RotationSequence=XYX  RotationSequenceAngles=[0 0 0]  RotationSequenceAnglesUnits=deg  RotationMatrix=[1 0 0; 0 1 0; 0 0 1]  Quaternion=[1 0 0 0]  TranslationMethod=Cartesian  TranslationCartesianOffset=[-166.59192436800632 39.825618202078182 -20.980989744703674]  TranslationCartesianOffsetUnits=mm  TranslationStandardAxis=+Z  TranslationStandardOffset=0  TranslationStandardOffsetUnits=mm  TranslationROffset=0  TranslationROffsetUnits=m  TranslationThetaOffset=0  TranslationThetaOffsetUnits=deg  TranslationZOffset=0  TranslationZOffsetUnits=m
  Transform3 : sm_lib/Frames and Transforms/Rigid Transform  RotationMethod=ArbitraryAxis  FollAlignAxisA=+X  BaseAlignAxisA=+Y  FollAlignAxisB=+Y  BaseAlignAxisB=+Z  RotationStandardAxis=+Z  RotationAngle=1.5707963267948968  RotationAngleUnits=rad  RotationArbitraryAxis=[0 1 0]  RotationSequenceAxes=FollowerAxes  RotationSequence=XYX  RotationSequenceAngles=[0 0 0]  RotationSequenceAnglesUnits=deg  RotationMatrix=[1 0 0; 0 1 0; 0 0 1]  Quaternion=[1 0 0 0]  TranslationMethod=Cartesian  TranslationCartesianOffset=[-166.59192436800632 39.825618202078182 -20.980989744703674]  TranslationCartesianOffsetUnits=mm  TranslationStandardAxis=+Z  TranslationStandardOffset=0  TranslationStandardOffsetUnits=mm  TranslationROffset=0  TranslationROffsetUnits=m  TranslationThetaOffset=0  TranslationThetaOffsetUnits=deg  TranslationZOffset=0  TranslationZOffsetUnits=m
  Transform4 : sm_lib/Frames and Transforms/Rigid Transform  RotationMethod=None  FollAlignAxisA=+X  BaseAlignAxisA=+Y  FollAlignAxisB=+Y  BaseAlignAxisB=+Z  RotationStandardAxis=+Z  RotationAngle=0  RotationAngleUnits=deg  RotationArbitraryAxis=[0 0 1]  RotationSequenceAxes=FollowerAxes  RotationSequence=XYX  RotationSequenceAngles=[0 0 0]  RotationSequenceAnglesUnits=deg  RotationMatrix=[1 0 0; 0 1 0; 0 0 1]  Quaternion=[1 0 0 0]  TranslationMethod=None  TranslationCartesianOffset=[0 0 0]  TranslationCartesianOffsetUnits=m  TranslationStandardAxis=+Z  TranslationStandardOffset=0  TranslationStandardOffsetUnits=m  TranslationROffset=0  TranslationROffsetUnits=m  TranslationThetaOffset=0  TranslationThetaOffsetUnits=deg  TranslationZOffset=0  TranslationZOffsetUnits=m
  Transform5 : sm_lib/Frames and Transforms/Rigid Transform  RotationMethod=ArbitraryAxis  FollAlignAxisA=+X  BaseAlignAxisA=+Y  FollAlignAxisB=+Y  BaseAlignAxisB=+Z  RotationStandardAxis=+Z  RotationAngle=3.1415926535897931  RotationAngleUnits=rad  RotationArbitraryAxis=[0 0.83121877946981937 -0.55594544755461728]  RotationSequenceAxes=FollowerAxes  RotationSequence=XYX  RotationSequenceAngles=[0 0 0]  RotationSequenceAnglesUnits=deg  RotationMatrix=[1 0 0; 0 1 0; 0 0 1]  Quaternion=[1 0 0 0]  TranslationMethod=Cartesian  TranslationCartesianOffset=[-333.18384873601264 5.2270863233389884 7.8152493791980202]  TranslationCartesianOffsetUnits=mm  TranslationStandardAxis=+Z  TranslationStandardOffset=0  TranslationStandardOffsetUnits=mm  TranslationROffset=0  TranslationROffsetUnits=m  TranslationThetaOffset=0  TranslationThetaOffsetUnits=deg  TranslationZOffset=0  TranslationZOffsetUnits=m
  Transform6 : sm_lib/Frames and Transforms/Rigid Transform  RotationMethod=ArbitraryAxis  FollAlignAxisA=+X  BaseAlignAxisA=+Y  FollAlignAxisB=+Y  BaseAlignAxisB=+Z  RotationStandardAxis=+Z  RotationAngle=1.5707963267948968  RotationAngleUnits=rad  RotationArbitraryAxis=[1 0 0]  RotationSequenceAxes=FollowerAxes  RotationSequence=XYX  RotationSequenceAngles=[0 0 0]  RotationSequenceAnglesUnits=deg  RotationMatrix=[1 0 0; 0 1 0; 0 0 1]  Quaternion=[1 0 0 0]  TranslationMethod=Cartesian  TranslationCartesianOffset=[-166.59192436800629 17.182941135267082 -24.98098974470367]  TranslationCartesianOffsetUnits=mm  TranslationStandardAxis=+Z  TranslationStandardOffset=0  TranslationStandardOffsetUnits=mm  TranslationROffset=0  TranslationROffsetUnits=m  TranslationThetaOffset=0  TranslationThetaOffsetUnits=deg  TranslationZOffset=0  TranslationZOffsetUnits=m
  Transform7 : sm_lib/Frames and Transforms/Rigid Transform  RotationMethod=ArbitraryAxis  FollAlignAxisA=+X  BaseAlignAxisA=+Y  FollAlignAxisB=+Y  BaseAlignAxisB=+Z  RotationStandardAxis=+Z  RotationAngle=1.0159852938148253  RotationAngleUnits=rad  RotationArbitraryAxis=[-1 0 0]  RotationSequenceAxes=FollowerAxes  RotationSequence=XYX  RotationSequenceAngles=[0 0 0]  RotationSequenceAnglesUnits=deg  RotationMatrix=[1 0 0; 0 1 0; 0 0 1]  Quaternion=[1 0 0 0]  TranslationMethod=Cartesian  TranslationCartesianOffset=[-172.59192436800629 90.586314327933948 3.4188407632840221]  TranslationCartesianOffsetUnits=mm  TranslationStandardAxis=+Z  TranslationStandardOffset=0  TranslationStandardOffsetUnits=mm  TranslationROffset=0  TranslationROffsetUnits=m  TranslationThetaOffset=0  TranslationThetaOffsetUnits=deg  TranslationZOffset=0  TranslationZOffsetUnits=m
  bras_1_RIGID : Subsystem
  palier_bras_1_RIGID : Subsystem
  palier_bras_2_RIGID : Subsystem
  F1 : PMIOPort  Side=Left
  F : PMIOPort  Port=2  Side=Right
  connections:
  Transform/LConn1 -- ReferenceFrame/RConn1 -- Transform6/LConn1 -- Transform7/LConn1 -- Transform5/LConn1 -- Transform4/LConn1 -- Transform3/LConn1 -- Transform2/LConn1 -- Transform1/LConn1
  Transform/RConn1 -- F/RConn1
  Transform1/RConn1 -- F1/RConn1
  Transform2/RConn1 -- bras_1_RIGID/LConn1
  AXE_BRAS_1_RIGID/LConn1 -- Transform3/RConn1
  Transform4/RConn1 -- palier_bras_1_RIGID/LConn1
  Transform5/RConn1 -- palier_bras_2_RIGID/LConn1
  Ressort_cable_1_RIGID/LConn1 -- Transform6/RConn1
  FIXATION_CABLE_1_RIGID/LConn1 -- Transform7/RConn1

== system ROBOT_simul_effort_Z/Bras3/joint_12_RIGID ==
  AXE_BRAS_1_RIGID : Subsystem
  ReferenceFrame : sm_lib/Frames and Transforms/Reference Frame
  Transform : sm_lib/Frames and Transforms/Rigid Transform  RotationMethod=ArbitraryAxis  FollAlignAxisA=+X  BaseAlignAxisA=+Y  FollAlignAxisB=+Y  BaseAlignAxisB=+Z  RotationStandardAxis=+Z  RotationAngle=2.2221940470110657  RotationAngleUnits=rad  RotationArbitraryAxis=[0.61437017396793003 -0.61437017396793026 0.49507431631749033]  RotationSequenceAxes=FollowerAxes  RotationSequence=XYX  RotationSequenceAngles=[0 0 0]  RotationSequenceAnglesUnits=deg  RotationMatrix=[1 0 0; 0 1 0; 0 0 1]  Quaternion=[1 0 0 0]  TranslationMethod=Cartesian  TranslationCartesianOffset=[-181.62772197331543 131.82453775326098 -130.42476989283941]  TranslationCartesianOffsetUnits=mm  TranslationStandardAxis=+Z  TranslationStandardOffset=0  TranslationStandardOffsetUnits=mm  TranslationROffset=0  TranslationROffsetUnits=m  TranslationThetaOffset=0  TranslationThetaOffsetUnits=deg  TranslationZOffset=0  TranslationZOffsetUnits=m
  Transform1 : sm_lib/Frames and Transforms/Rigid Transform  RotationMethod=ArbitraryAxis  FollAlignAxisA=+X  BaseAlignAxisA=+Y  FollAlignAxisB=+Y  BaseAlignAxisB=+Z  RotationStandardAxis=+Z  RotationAngle=2.0943951023931953  RotationAngleUnits=rad  RotationArbitraryAxis=[0.57735026918962595 0.57735026918962584 0.57735026918962562]  RotationSequenceAxes=FollowerAxes  RotationSequence=XYX  RotationSequenceAngles=[0 0 0]  RotationSequenceAnglesUnits=deg  RotationMatrix=[1 0 0; 0 1 0; 0 0 1]  Quaternion=[1 0 0 0]  TranslationMethod=Cartesian  TranslationCartesianOffset=[-177.62772197331262 126.39913469758682 -143.11837070913361]  TranslationCartesianOffsetUnits=mm  TranslationStandardAxis=+Z  TranslationStandardOffset=0  TranslationStandardOffsetUnits=mm  TranslationROffset=0  TranslationROffsetUnits=m  TranslationThetaOffset=0  TranslationThetaOffsetUnits=deg  TranslationZOffset=0  TranslationZOffsetUnits=m
  Transform2 : sm_lib/Frames and Transforms/Rigid Transform  RotationMethod=ArbitraryAxis  FollAlignAxisA=+X  BaseAlignAxisA=+Y  FollAlignAxisB=+Y  BaseAlignAxisB=+Z  RotationStandardAxis=+Z  RotationAngle=2.2221940470110662  RotationAngleUnits=rad  RotationArbitraryAxis=[0.61437017396793026 -0.61437017396793059 0.49507431631748977]  RotationSequenceAxes=FollowerAxes  RotationSequence=XYX  RotationSequenceAngles=[0 0 0]  RotationSequenceAnglesUnits=deg  RotationMatrix=[1 0 0; 0 1 0; 0 0 1]  Quaternion=[1 0 0 0]  TranslationMethod=Cartesian  TranslationCartesianOffset=[-153.62772197331537 131.82453775326132 -130.4247698928408]  TranslationCartesianOffsetUnits=mm  TranslationStandardAxis=+Z  TranslationStandardOffset=0  TranslationStandardOffsetUnits=mm  TranslationROffset=0  TranslationROffsetUnits=m  TranslationThetaOffset=0  TranslationThetaOffsetUnits=deg  TranslationZOffset=0  TranslationZOffsetUnits=m
  Transform3 : sm_lib/Frames and Transforms/Rigid Transform  RotationMethod=ArbitraryAxis  FollAlignAxisA=+X  BaseAlignAxisA=+Y  FollAlignAxisB=+Y  BaseAlignAxisB=+Z  RotationStandardAxis=+Z  RotationAngle=1.7850283121554718  RotationAngleUnits=rad  RotationArbitraryAxis=[1 8.3181277610745589e-16 -6.6018680201685363e-16]  RotationSequenceAxes=FollowerAxes  RotationSequence=XYX  RotationSequenceAngles=[0 0 0]  RotationSequenceAnglesUnits=deg  RotationMatrix=[1 0 0; 0 1 0; 0 0 1]  Quaternion=[1 0 0 0]  TranslationMethod=Cartesian  TranslationCartesianOffset=[-167.62772197331242 128.0999109638598 -150.93549038919824]  TranslationCartesianOffsetUnits=mm  TranslationStandardAxis=+Z  TranslationStandardOffset=0  TranslationStandardOffsetUnits=mm  TranslationROffset=0  TranslationROffsetUnits=m  TranslationThetaOffset=0  TranslationThetaOffsetUnits=deg  TranslationZOffset=0  TranslationZOffsetUnits=m
  Transform4 : sm_lib/Frames and Transforms/Rigid Transform  RotationMethod=ArbitraryAxis  FollAlignAxisA=+X  BaseAlignAxisA=+Y  FollAlignAxisB=+Y  BaseAlignAxisB=+Z  RotationStandardAxis=+Z  RotationAngle=1.5707963267948968  RotationAngleUnits=rad  RotationArbitraryAxis=[5.5511151231257809e-17 -1 -5.5511151231257809e-17]  RotationSequenceAxes=FollowerAxes  RotationSequence=XYX  RotationSequenceAngles=[0 0 0]  RotationSequenceAnglesUnits=deg  RotationMatrix=[1 0 0; 0 1 0; 0 0 1]  Quaternion=[1 0 0 0]  TranslationMethod=Cartesian  TranslationCartesianOffset=[-167.62772197331242 126.39913469761733 -143.11837070915067]  TranslationCartesianOffsetUnits=mm  TranslationStandardAxis=+Z  TranslationStandardOffset=0  TranslationStandardOffsetUnits=mm  TranslationROffset=0  TranslationROffsetUnits=m  TranslationThetaOffset=0  TranslationThetaOffsetUnits=deg  TranslationZOffset=0  TranslationZOffsetUnits=m
  joint_1_RIGID : Subsystem
  F2 : PMIOPort  Side=Right
  F1 : PMIOPort  Port=2  Side=Left
  F : PMIOPort  Port=3  Side=Right
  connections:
  Transform/LConn1 -- ReferenceFrame/RConn1 -- Transform3/LConn1 -- Transform4/LConn1 -- Transform2/LConn1 -- Transform1/LConn1
  Transform/RConn1 -- F/RConn1
  Transform1/RConn1 -- F1/RConn1
  Transform2/RConn1 -- F2/RConn1
  Transform3/RConn1 -- joint_1_RIGID/LConn1
  AXE_BRAS_1_RIGID/LConn1 -- Transform4/RConn1

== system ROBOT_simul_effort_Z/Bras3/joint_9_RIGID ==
  AXE_BRAS_1_RIGID : Subsystem
  ReferenceFrame : sm_lib/Frames and Transforms/Reference Frame
  Transform : sm_lib/Frames and Transforms/Rigid Transform  RotationMethod=ArbitraryAxis  FollAlignAxisA=+X  BaseAlignAxisA=+Y  FollAlignAxisB=+Y  BaseAlignAxisB=+Z  RotationStandardAxis=+Z  RotationAngle=1.9754511492118274  RotationAngleUnits=rad  RotationArbitraryAxis=[-0.53149434051907796 -0.53149434051907751 -0.65956616953295999]  RotationSequenceAxes=FollowerAxes  RotationSequence=XYX  RotationSequenceAngles=[0 0 0]  RotationSequenceAnglesUnits=deg  RotationMatrix=[1 0 0; 0 1 0; 0 0 1]  Quaternion=[1 0 0 0]  TranslationMethod=Cartesian  TranslationCartesianOffset=[-181.62772197330938 116.19029839316687 -133.82632242532907]  TranslationCartesianOffsetUnits=mm  TranslationStandardAxis=+Z  TranslationStandardOffset=0  TranslationStandardOffsetUnits=mm  TranslationROffset=0  TranslationROffsetUnits=m  TranslationThetaOffset=0  TranslationThetaOffsetUnits=deg  TranslationZOffset=0  TranslationZOffsetUnits=m
  Transform1 : sm_lib/Frames and Transforms/Rigid Transform  RotationMethod=ArbitraryAxis  FollAlignAxisA=+X  BaseAlignAxisA=+Y  FollAlignAxisB=+Y  BaseAlignAxisB=+Z  RotationStandardAxis=+Z  RotationAngle=2.0943951023931993  RotationAngleUnits=rad  RotationArbitraryAxis=[0.57735026918962373 0.57735026918962706 0.57735026918962651]  RotationSequenceAxes=FollowerAxes  RotationSequence=XYX  RotationSequenceAngles=[0 0 0]  RotationSequenceAnglesUnits=deg  RotationMatrix=[1 0 0; 0 1 0; 0 0 1]  Quaternion=[1 0 0 0]  TranslationMethod=Cartesian  TranslationCartesianOffset=[-188.74209771778101 126.39913469761137 -143.11837070916158]  TranslationCartesianOffsetUnits=mm  TranslationStandardAxis=+Z  TranslationStandardOffset=0  TranslationStandardOffsetUnits=mm  TranslationROffset=0  TranslationROffsetUnits=m  TranslationThetaOffset=0  TranslationThetaOffsetUnits=deg  TranslationZOffset=0  TranslationZOffsetUnits=m
  Transform2 : sm_lib/Frames and Transforms/Rigid Transform  RotationMethod=ArbitraryAxis  FollAlignAxisA=+X  BaseAlignAxisA=+Y  FollAlignAxisB=+Y  BaseAlignAxisB=+Z  RotationStandardAxis=+Z  RotationAngle=1.9754511492118267  RotationAngleUnits=rad  RotationArbitraryAxis=[-0.53149434051907773 -0.53149434051907751 -0.6595661695329601]  RotationSequenceAxes=FollowerAxes  RotationSequence=XYX  RotationSequenceAngles=[0 0 0]  RotationSequenceAnglesUnits=deg  RotationMatrix=[1 0 0; 0 1 0; 0 0 1]  Quaternion=[1 0 0 0]  TranslationMethod=Cartesian  TranslationCartesianOffset=[-153.62772197330932 116.19029839316653 -133.82632242532716]  TranslationCartesianOffsetUnits=mm  TranslationStandardAxis=+Z  TranslationStandardOffset=0  TranslationStandardOffsetUnits=mm  TranslationROffset=0  TranslationROffsetUnits=m  TranslationThetaOffset=0  TranslationThetaOffsetUnits=deg  TranslationZOffset=0  TranslationZOffsetUnits=m
  Transform3 : sm_lib/Frames and Transforms/Rigid Transform  RotationMethod=ArbitraryAxis  FollAlignAxisA=+X  BaseAlignAxisA=+Y  FollAlignAxisB=+Y  BaseAlignAxisB=+Z  RotationStandardAxis=+Z  RotationAngle=1.785028312155472  RotationAngleUnits=rad  RotationArbitraryAxis=[1 8.002259724525313e-16 -6.8382944364994947e-16]  RotationSequenceAxes=FollowerAxes  RotationSequence=XYX  RotationSequenceAngles=[0 0 0]  RotationSequenceAnglesUnits=deg  RotationMatrix=[1 0 0; 0 1 0; 0 0 1]  Quaternion=[1 0 0 0]  TranslationMethod=Cartesian  TranslationCartesianOffset=[-167.62772197331239 128.09991096385986 -150.93549038919818]  TranslationCartesianOffsetUnits=mm  TranslationStandardAxis=+Z  TranslationStandardOffset=0  TranslationStandardOffsetUnits=mm  TranslationROffset=0  TranslationROffsetUnits=m  TranslationThetaOffset=0  TranslationThetaOffsetUnits=deg  TranslationZOffset=0  TranslationZOffsetUnits=m
  Transform4 : sm_lib/Frames and Transforms/Rigid Transform  RotationMethod=ArbitraryAxis  FollAlignAxisA=+X  BaseAlignAxisA=+Y  FollAlignAxisB=+Y  BaseAlignAxisB=+Z  RotationStandardAxis=+Z  RotationAngle=1.5707963267948968  RotationAngleUnits=rad  RotationArbitraryAxis=[-0 -1 -0]  RotationSequenceAxes=FollowerAxes  RotationSequence=XYX  RotationSequenceAngles=[0 0 0]  RotationSequenceAnglesUnits=deg  RotationMatrix=[1 0 0; 0 1 0; 0 0 1]  Quaternion=[1 0 0 0]  TranslationMethod=Cartesian  TranslationCartesianOffset=[-167.62772197331236 126.39913469761737 -143.11837070915064]  TranslationCartesianOffsetUnits=mm  TranslationStandardAxis=+Z  TranslationStandardOffset=0  TranslationStandardOffsetUnits=mm  TranslationROffset=0  TranslationROffsetUnits=m  TranslationThetaOffset=0  TranslationThetaOffsetUnits=deg  TranslationZOffset=0  TranslationZOffsetUnits=m
  joint_1_RIGID : Subsystem
  F2 : PMIOPort  Side=Left
  F : PMIOPort  Port=2  Side=Left
  F1 : PMIOPort  Port=3  Side=Right
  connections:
  Transform/LConn1 -- ReferenceFrame/RConn1 -- Transform3/LConn1 -- Transform4/LConn1 -- Transform2/LConn1 -- Transform1/LConn1
  Transform/RConn1 -- F/RConn1
  Transform1/RConn1 -- F1/RConn1
  Transform2/RConn1 -- F2/RConn1
  Transform3/RConn1 -- joint_1_RIGID/LConn1
  AXE_BRAS_1_RIGID/LConn1 -- Transform4/RConn1
